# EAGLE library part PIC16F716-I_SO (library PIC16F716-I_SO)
Micro 16b, 3.5 KB Flash, PIC16F716-I/SO Source: Datasheet
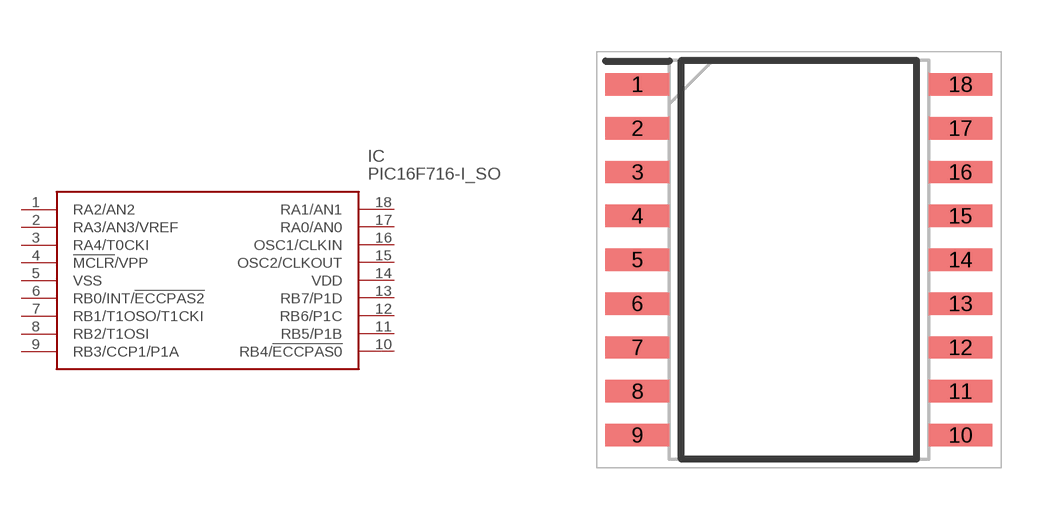
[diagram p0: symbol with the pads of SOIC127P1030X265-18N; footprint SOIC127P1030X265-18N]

Designator prefix IC

## PIC16F716-I_SO (Description: Micro 16b, 3.5 KB Flash, PIC16F716-I/SO; Height: 2.65mm; Manufacturer_Name: Microchip; Manufacturer_Part_Number: PIC16F716-I/SO; Mouser_Part_Number: 579-PIC16F716-I/SO; Mouser_Price-Stock: https://www.mouser.co.uk/ProductDetail/Microchip-Technology/PIC16F716-I-SO?qs=z30FE1aq6wZ1zisuoVAr%2FQ%3D%3D)  [SOIC127P1030X265-18N]
1  RA2/AN2
2  RA3/AN3/VREF
3  RA4/T0CKI
4  !MCLR!/VPP
5  VSS
6  RB0/INT/!ECCPAS2
7  RB1/T1OSO/T1CKI
8  RB2/T1OSI
9  RB3/CCP1/P1A
10  RB4/!ECCPAS0
11  RB5/P1B
12  RB6/P1C
13  RB7/P1D
14  VDD
15  OSC2/CLKOUT
16  OSC1/CLKIN
17  RA0/AN0
18  RA1/AN1

## Footprint SOIC127P1030X265-18N (pad centres in mm)
PIC16F716-I/SO-1
smd 1.85 x 0.65: 1 -4.675,5.08; 2 -4.675,3.81; 3 -4.675,2.54; 4 -4.675,1.27; 5 -4.675,0; 6 -4.675,-1.27; 7 -4.675,-2.54; 8 -4.675,-3.81; 9 -4.675,-5.08; 10 4.675,-5.08; 11 4.675,-3.81; 12 4.675,-2.54; 13 4.675,-1.27; 14 4.675,0; 15 4.675,1.27; 16 4.675,2.54; 17 4.675,3.81; 18 4.675,5.08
